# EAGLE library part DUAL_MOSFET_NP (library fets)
MOSFET N/P-CH 20V 2A 6-TSOP
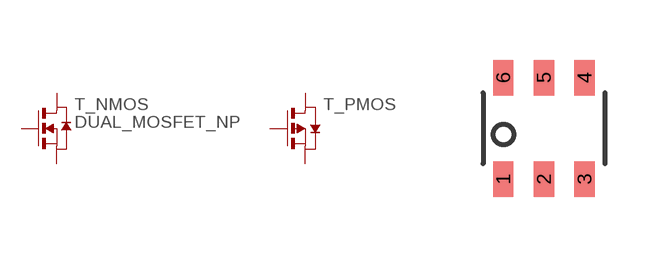
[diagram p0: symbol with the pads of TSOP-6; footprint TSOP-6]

Designator prefix T; gates _NMOS=N_MOSFET _PMOS=P_MOSFET

## DUAL_MOSFET_NP (DIGIKEY: SI3585DV-T1-E3CT-ND)  [TSOP-6]
1  _NMOS:G  pas
2  _PMOS:S  pas
3  _PMOS:G  pas
4  _PMOS:D  pas
5  _NMOS:S  pas
6  _NMOS:D  pas

## Footprint TSOP-6 (pad centres in mm)
smd 0.508 x 0.889: 1 -1.016,-1.27; 2 0,-1.27; 3 1.016,-1.27; 4 1.016,1.27; 5 0,1.27; 6 -1.016,1.27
